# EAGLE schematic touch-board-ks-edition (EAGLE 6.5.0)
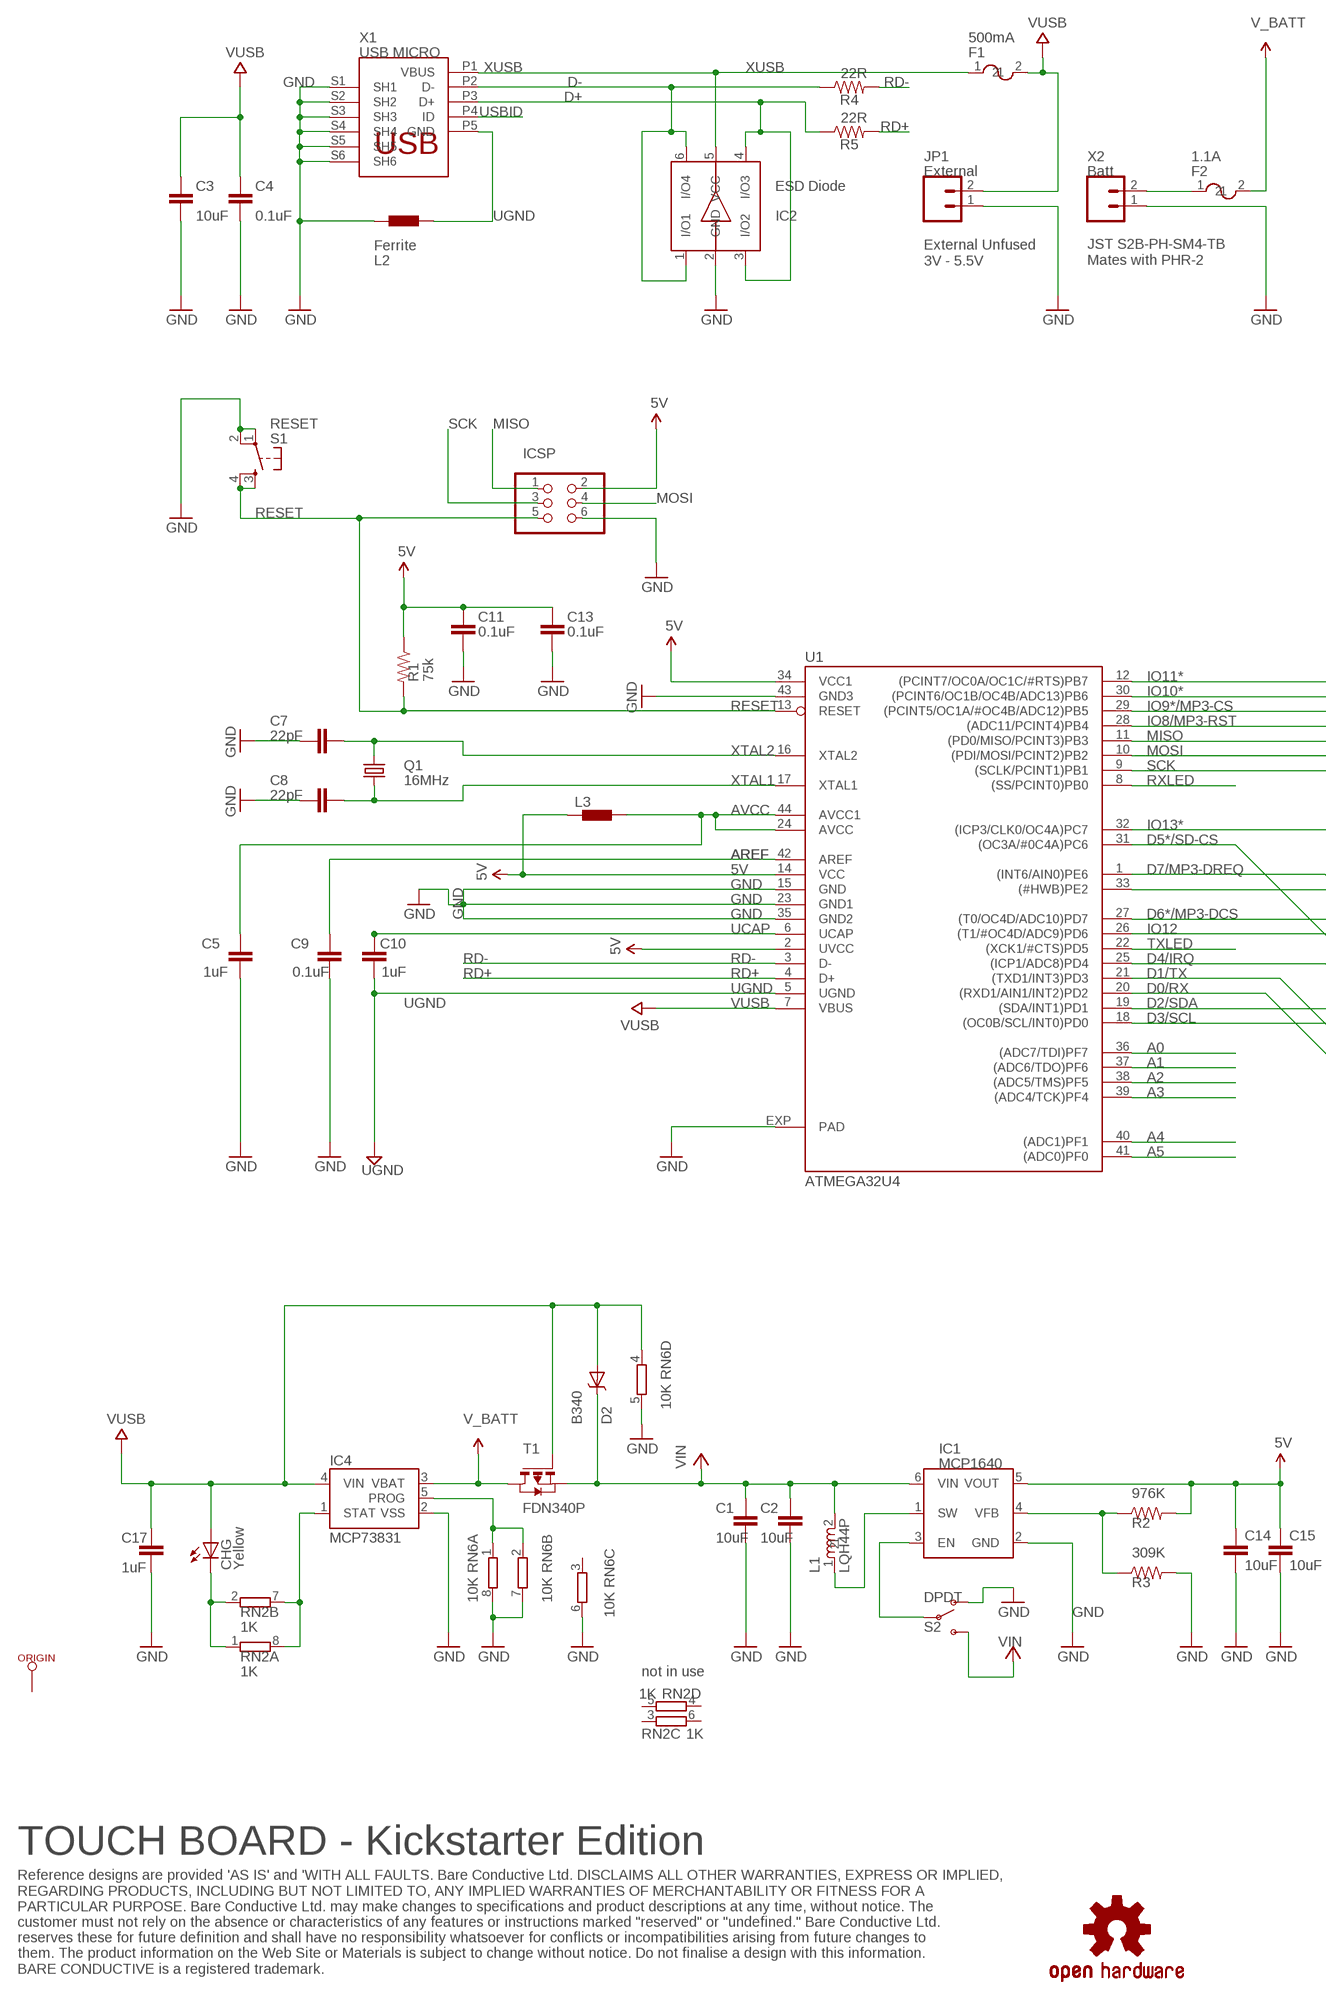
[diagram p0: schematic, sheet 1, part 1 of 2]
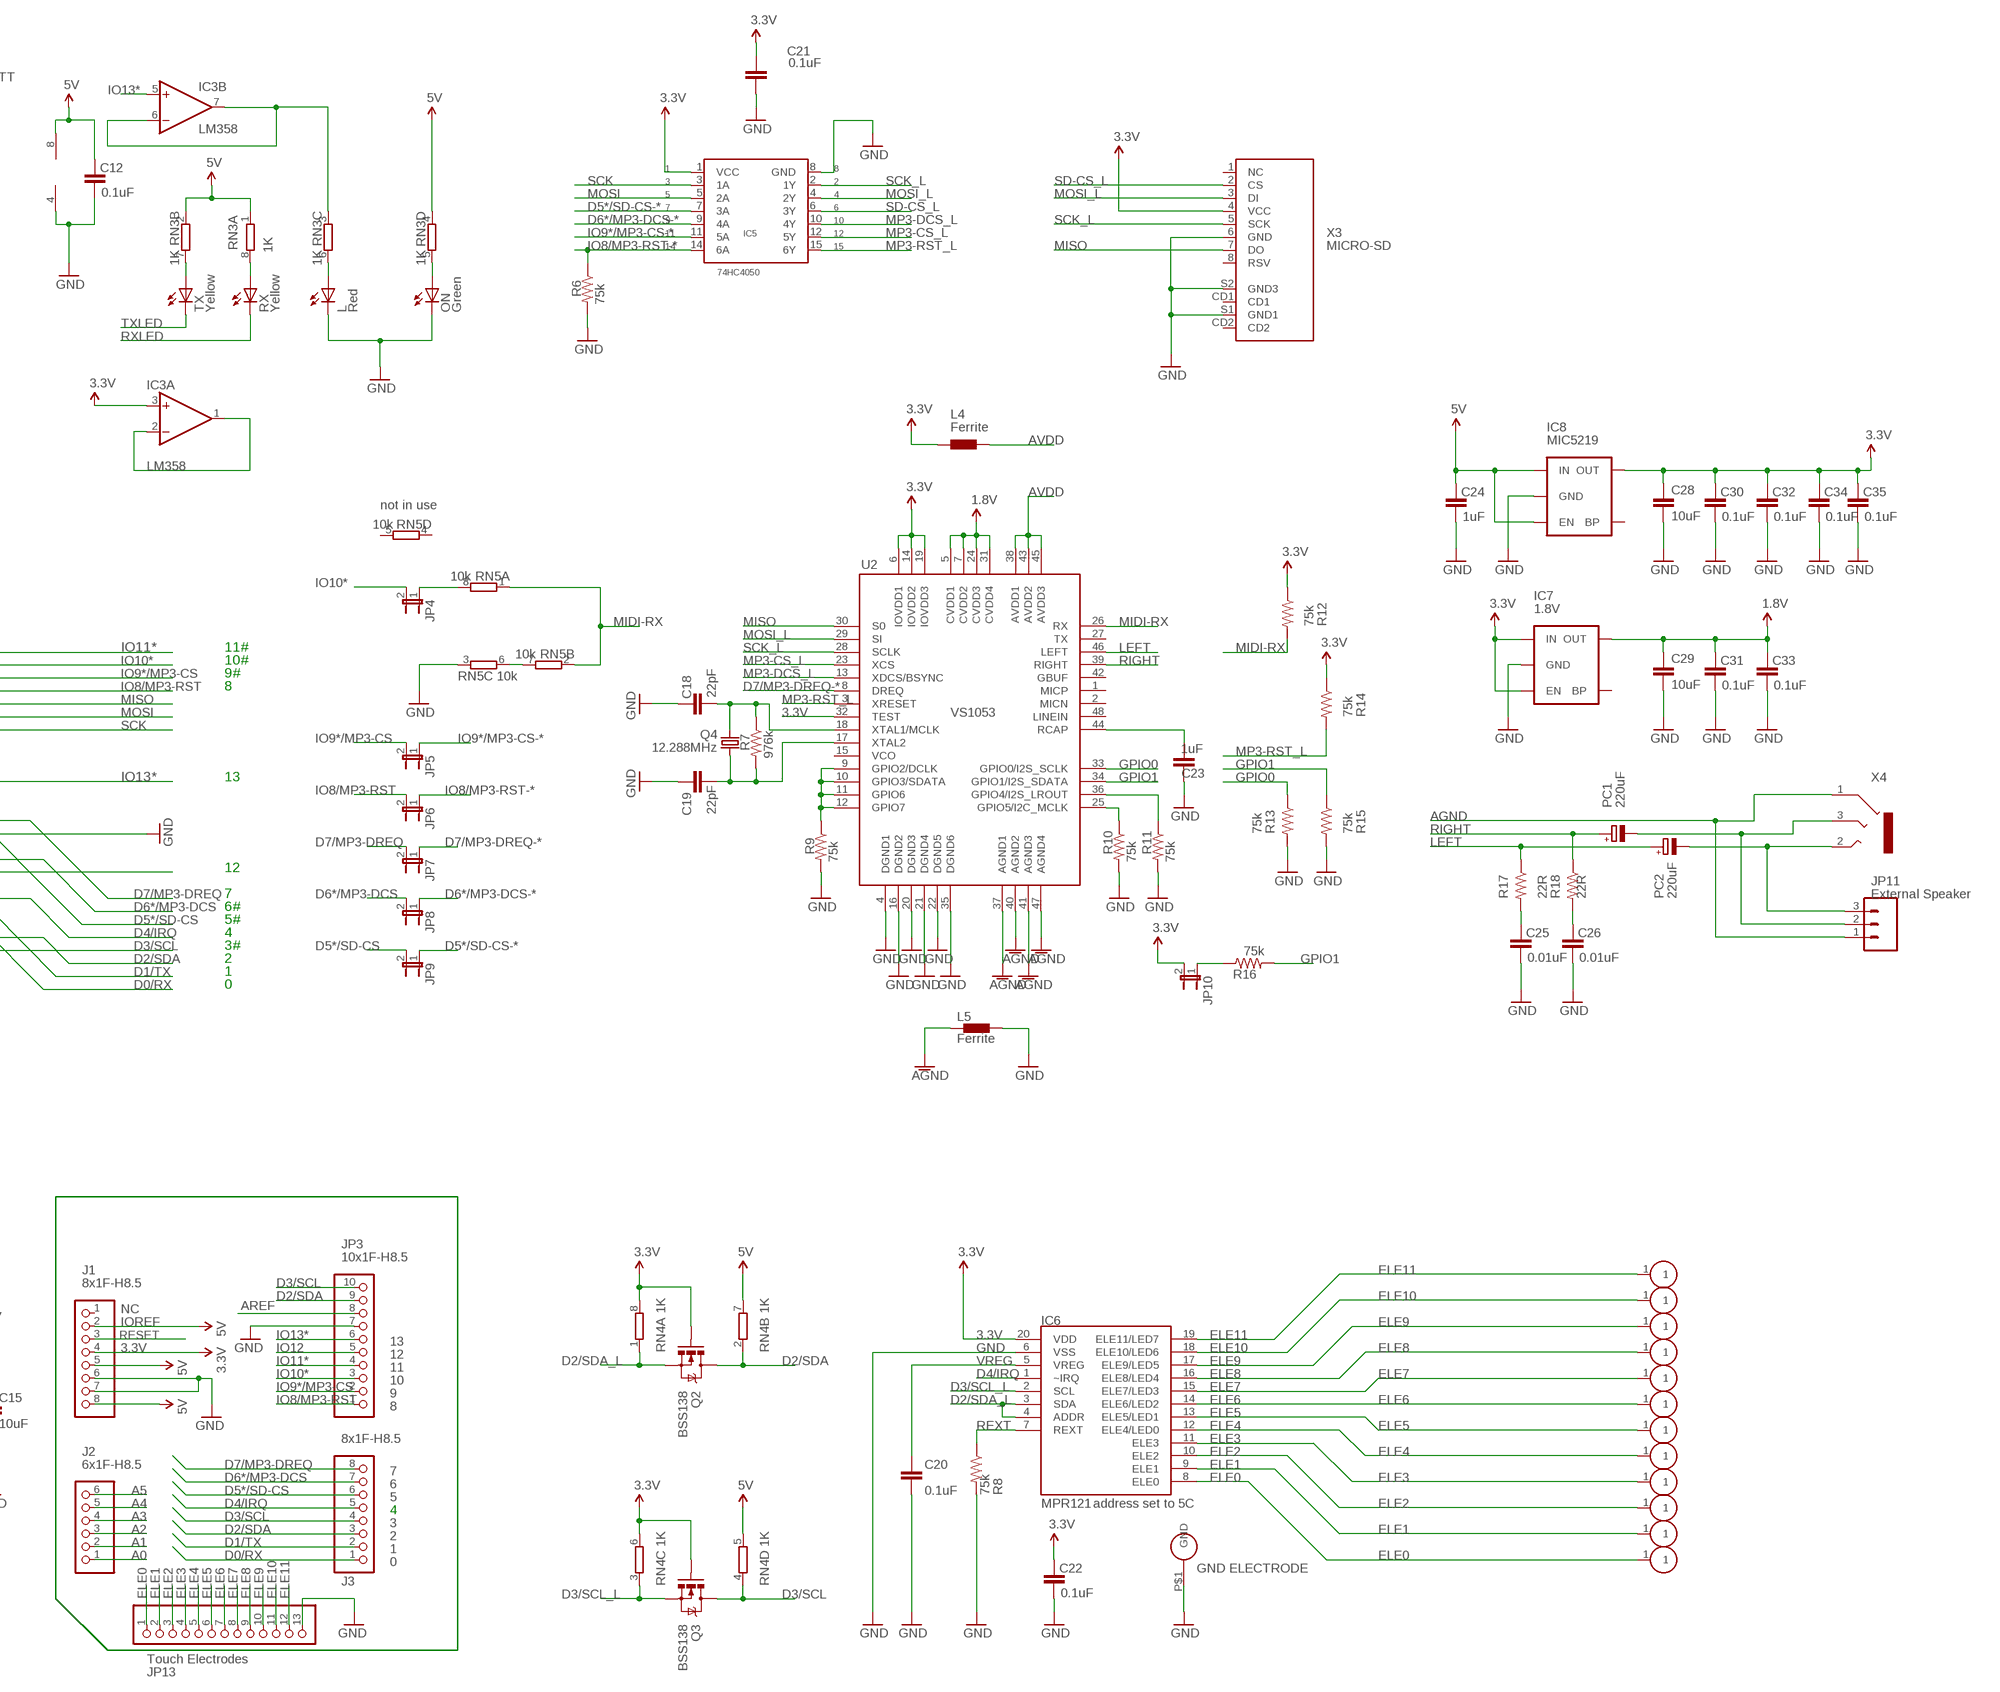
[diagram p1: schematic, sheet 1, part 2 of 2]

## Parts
C1  10uF  CAP1206  [1206]
C2  10uF  CAP1206  [1206]
C3  10uF  CAP1206  [1206]
C4  0.1uF  CAP0402-CAP  [0402-CAP]
C5  1uF  CAP0402-CAP  [0402-CAP]
C7  22pF  CAP0402-CAP  [0402-CAP]
C8  22pF  CAP0402-CAP  [0402-CAP]
C9  0.1uF  CAP0402-CAP  [0402-CAP]
C10  1uF  CAP0402-CAP  [0402-CAP]
C11  0.1uF  CAP0402-CAP  [0402-CAP]
C12  0.1uF  CAP0402-CAP  [0402-CAP]
C13  0.1uF  CAP0402-CAP  [0402-CAP]
C14  10uF  CAP1206  [1206]
C15  10uF  CAP1206  [1206]
C17  1uF  CAP0402-CAP  [0402-CAP]
C18  22pF  CAP0402-CAP  [0402-CAP]
C19  22pF  CAP0402-CAP  [0402-CAP]
C20  0.1uF  CAP0402-CAP  [0402-CAP]
C21  0.1uF  CAP0402-CAP  [0402-CAP]
C22  0.1uF  CAP0402-CAP  [0402-CAP]
C23  1uF  CAP0402-CAP  [0402-CAP]
C24  1uF  CAP0402-CAP  [0402-CAP]
C25  0.01uF  CAP0402-CAP  [0402-CAP]
C26  0.01uF  CAP0402-CAP  [0402-CAP]
C28  10uF  CAP1206  [1206]
C29  10uF  CAP1206  [1206]
C30  0.1uF  CAP0402-CAP  [0402-CAP]
C31  0.1uF  CAP0402-CAP  [0402-CAP]
C32  0.1uF  CAP0402-CAP  [0402-CAP]
C33  0.1uF  CAP0402-CAP  [0402-CAP]
C34  0.1uF  CAP0402-CAP  [0402-CAP]
C35  0.1uF  CAP0402-CAP  [0402-CAP]
CHG  Yellow  LEDCHIPLED_0805  [CHIPLED_0805]
D2  B340  DIODE-SCHOTTKY_  [SMA-DIODE]
F1  500mA  PTC  [0805]
F2  1.1A  PTC  [0805]
IC1  MCP1640  BOOST-REG  [6-LEAD-SOT23]
IC2  ESD Diode  PRTR5V  [SOT457]
IC3  LM358  LMV358MMX  [MSOP08]
IC4  MCP73831  [SOT23-5]
IC5  74HC4050  74HC4050PW  [TSSOP-16]
IC6  MPR121  MPR121QFN20  [QFN-20-0.4MM]
IC7  1.8V  V_REG_LDOSMD2  [SC70]
IC8  MIC5219  V_REG_LDOSMD  [SOT23-5]
ICSP  ICSP  PINHD-2X3  [2X03]
J1  8x1F-H8.5  PINHD-1X8  [1X08]
J2  6x1F-H8.5  PINHD-1X6  [1X06]
J3  8x1F-H8.5  PINHD-1X8  [1X08]
JP1  External  M02PTH  [1X02]
JP3  10x1F-H8.5  PINHD-1X10  [1X10]
JP4  JUMPER-2SMD-NO  [SJ_2S-NO]
JP5  JUMPER-2SMD-NC  [SJ_2S]
JP6  JUMPER-2SMD-NC  [SJ_2S]
JP7  JUMPER-2SMD-NC  [SJ_2S]
JP8  JUMPER-2SMD-NC  [SJ_2S]
JP9  JUMPER-2SMD-NC  [SJ_2S]
JP10  JUMPER-2SMD-NO  [SJ_2S-NO]
JP11  External Speaker  M03PTH  [1X03]
JP13  Touch Electrodes  PINHD-1X13  [1X13]
L  Red  LEDCHIPLED_0805  [CHIPLED_0805]
L1  LQH44P  [LQH44PN100MP0L]
L2  Ferrite  BLM15HB121SN1  [0402]
L3  BLM15HB121SN1  [0402]
L4  Ferrite  BLM15HB121SN1  [0402]
L5  Ferrite  BLM15HB121SN1  [0402]
ON  Green  LEDCHIPLED_0805  [CHIPLED_0805]
ORIGIN  TP_SP  [TP-SP]
PC1  220uF  CPOL-EUD  [PANASONIC_D]
PC2  220uF  CPOL-EUD  [PANASONIC_D]
Q1  16MHz  CRYSTAL5X3  [CRYSTAL-SMD-5X3]
Q2  BSS138  MOSFET-NCHANNELSMD  [SOT23-3]
Q3  BSS138  MOSFET-NCHANNELSMD  [SOT23-3]
Q4  12.288MHz  CRYSTAL5X3  [CRYSTAL-SMD-5X3]
R1  75k  RESISTOR0402-RES  [0402-RES]
R2  976K  RESISTOR0402-RES  [0402-RES]
R3  309K  RESISTOR0402-RES  [0402-RES]
R4  22R  RESISTOR0402-RES  [0402-RES]
R5  22R  RESISTOR0402-RES  [0402-RES]
R6  75k  RESISTOR0402-RES  [0402-RES]
R7  976k  RESISTOR0402-RES  [0402-RES]
R8  75k  RESISTOR0402-RES  [0402-RES]
R9  75k  RESISTOR0402-RES  [0402-RES]
R10  75k  RESISTOR0402-RES  [0402-RES]
R11  75k  RESISTOR0402-RES  [0402-RES]
R12  75k  RESISTOR0402-RES  [0402-RES]
R13  75k  RESISTOR0402-RES  [0402-RES]
R14  75k  RESISTOR0402-RES  [0402-RES]
R15  75k  RESISTOR0402-RES  [0402-RES]
R16  75k  RESISTOR0402-RES  [0402-RES]
R17  22R  RESISTOR0402-RES  [0402-RES]
R18  22R  RESISTOR0402-RES  [0402-RES]
RN2  1K  4R-NCAY16  [CAY16]
RN3  1K  4R-NCAY16  [CAY16]
RN4  1K  4R-NCAY16  [CAY16]
RN5  10k  4R-NCAY16  [CAY16]
RN6  10K  4R-NCAY16  [CAY16]
RX  Yellow  LEDCHIPLED_0805  [CHIPLED_0805]
S1  RESET  TAC_SWITCHSND  [TACTILE_SWITCH_SMD@1]
S2  DPDT  DPDT-SWITCH  [JS202011SCQN]
T1  FDN340P  PMOSSOT23  [SOT-23]
TX  Yellow  LEDCHIPLED_0805  [CHIPLED_0805]
U1  ATMEGA32U4  ATMEGA32U4-XUMU  [QFN44ML7X7]
U2  VS1053  VS1033  [LQFP-48]
U$1  EDGE-ELEC-LEFT  [EDGE-ELEC-LEFT]
U$3  EDGE-ELEC-RIGHT  [EDGE-ELEC-RIGHT]
U$6  EDGE-GND  [EDGE-GND]
U$8  OSHW-LOGO  [OSHW-LOGO]
U$17  EDGE-ELEC  [EDGE-ELEC]
U$18  EDGE-ELEC  [EDGE-ELEC]
U$22  EDGE-ELEC  [EDGE-ELEC]
U$24  EDGE-ELEC  [EDGE-ELEC]
U$26  EDGE-ELEC  [EDGE-ELEC]
U$27  EDGE-ELEC  [EDGE-ELEC]
U$28  EDGE-ELEC  [EDGE-ELEC]
U$29  EDGE-ELEC  [EDGE-ELEC]
U$30  EDGE-ELEC  [EDGE-ELEC]
U$31  EDGE-ELEC  [EDGE-ELEC]
X1  USB MICRO  MYCON2_USB-MINI-B  [CON2_USB_MICRO_B_AT]
X2  Batt  M02-JST-2MM-SMT  [JST-2-SMD]
X3  MICRO-SD  TOBY-SD  [MSDC-PP-02]
X4  SJ-3523  [3POLE-JACK]

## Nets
1.8V: C29.1 C31.2 C33.2 IC7.5(OUT) U2.5(CVDD1) U2.7(CVDD2) U2.24(CVDD3) U2.31(CVDD4)
3.3V: C21.2 C22.2 C28.1 C30.2 C32.2 C34.2 C35.2 IC3.3(A:+IN) IC5.1(VCC) IC6.20(VDD) IC7.1(IN) IC7.3(EN) IC8.5(OUT) J1.4 JP10.2 L4.1 Q2.1(G) Q3.1(G) R12.1 R14.1 RN4.6 RN4.8 U2.6(IOVDD1) U2.14(IOVDD2) U2.19(IOVDD3) U2.32(TEST) X3.4(VCC)
5V: C11.2 C12.2 C13.2 C14.1 C15.1 C24.2 IC1.5(VOUT) IC3.8(P:V+) IC8.1(IN) IC8.3(EN) ICSP.2 J1.2 J1.5 J1.8 L3.1 R1.1 R2.2 RN3.1 RN3.2 RN3.4 RN4.5 RN4.7 U1.2(UVCC) U1.14(VCC) U1.34(VCC1)
A0: J2.1 U1.36((ADC7/TDI)PF7)
A1: J2.2 U1.37((ADC6/TDO)PF6)
A2: J2.3 U1.38((ADC5/TMS)PF5)
A3: J2.4 U1.39((ADC4/TCK)PF4)
A4: J2.5 U1.40((ADC1)PF1)
A5: J2.6 U1.41((ADC0)PF0)
AGND: JP11.1 L5.1 U2.37(AGND1) U2.40(AGND2) U2.41(AGND3) U2.47(AGND4) X4.1
AREF [aref]: C9.2 JP3.8 U1.42(AREF)
AVCC: C5.2 L3.2 U1.24(AVCC) U1.44(AVCC1)
AVDD: L4.2 U2.38(AVDD1) U2.43(AVDD2) U2.45(AVDD3)
D0/RX: J3.1 U1.20((RXD1/AIN1/INT2)PD2)
D1/TX: J3.2 U1.21((TXD1/INT3)PD3)
D2/SDA: J3.3 JP3.9 Q2.3(D) RN4.2 U1.19((SDA/INT1)PD1)
D2/SDA_L: IC6.3(SDA) IC6.4(ADDR) Q2.2(S) RN4.1
D3/SCL: J3.4 JP3.10 Q3.3(D) RN4.4 U1.18((OC0B/SCL/INT0)PD0)
D3/SCL_L: IC6.2(SCL) Q3.2(S) RN4.3
D4/IRQ: IC6.1(~IRQ) J3.5 U1.25((ICP1/ADC8)PD4)
D5*/SD-CS: J3.6 JP9.2 U1.31((OC3A/#0C4A)PC6)
D5*/SD-CS-*: IC5.7(3A) JP9.1
D6*/MP3-DCS: J3.7 JP8.2 U1.27((T0/OC4D/ADC10)PD7)
D6*/MP3-DCS-*: IC5.9(4A) JP8.1
D7/MP3-DREQ: J3.8 JP7.2 U1.1((INT6/AIN0)PE6)
D7/MP3-DREQ-*: JP7.1 U2.8(DREQ)
D+: IC2.3(I/O2) IC2.4(I/O3) R5.1 X1.P3(D+)
D-: IC2.1(I/O1) IC2.6(I/O4) R4.1 X1.P2(D-)
ELE0: IC6.8(ELE0) JP13.1 U$1.1
ELE1: IC6.9(ELE1) JP13.2 U$31.1
ELE2: IC6.10(ELE2) JP13.3 U$30.1
ELE3: IC6.11(ELE3) JP13.4 U$29.1
ELE4: IC6.12(ELE4/LED0) JP13.5 U$28.1
ELE5: IC6.13(ELE5/LED1) JP13.6 U$27.1
ELE6: IC6.14(ELE6/LED2) JP13.7 U$26.1
ELE7: IC6.15(ELE7/LED3) JP13.8 U$24.1
ELE8: IC6.16(ELE8/LED4) JP13.9 U$22.1
ELE9: IC6.17(ELE9/LED5) JP13.10 U$18.1
ELE10: IC6.18(ELE10/LED6) JP13.11 U$17.1
ELE11: IC6.19(ELE11/LED7) JP13.12 U$3.1
G1: R9.1 U2.9(GPIO2/DCLK) U2.10(GPIO3/SDATA) U2.11(GPIO6) U2.12(GPIO7)
G2: R10.1 U2.25(GPIO5/I2C_MCLK)
GND [gnd]: C1.2 C2.2 C3.2 C4.1 C5.1 C7.2 C8.2 C9.1 C11.1 C12.1 C13.1 C14.2 C15.2 C17.1 C18.2 C19.2 C20.1 C21.1 C22.1 C23.2 C24.1 C25.1 C26.1 C28.2 C29.2 C30.1 C31.1 C32.1 C33.1 C34.1 C35.1 IC1.2(GND) IC2.2(GND) IC3.4(P:V-) IC4.2(VSS) IC5.8(GND) IC6.6(VSS) IC7.2(GND) IC8.2(GND) ICSP.6 J1.6 J1.7 JP1.1 JP3.7 JP13.13 L2.1 L5.2 L.C ON.C R3.2 R6.2 R8.2 R9.2 R10.2 R11.2 R13.2 R15.2 RN5.3 RN6.5 RN6.6 RN6.7 RN6.8 S1.1 S1.2 S2.4 U1.15(GND) U1.23(GND1) U1.33((#HWB)PE2) U1.35(GND2) U1.43(GND3) U1.EXP(PAD) U2.4(DGND1) U2.16(DGND2) U2.20(DGND3) U2.21(DGND4) U2.22(DGND5) U2.35(DGND6) U$6.P$1(GND) X1.S1(SH1) X1.S2(SH2) X1.S3(SH3) X1.S4(SH4) X1.S5(SH5) X1.S6(SH6) X2.1 X3.6(GND) X3.S1(GND1) X3.S2(GND3)
GPIO0: R13.1 U2.33(GPIO0/I2S_SCLK)
GPIO1: R15.1 R16.2 U2.34(GPIO1/I2S_SDATA)
IO8/MP3-RST: JP3.1 JP6.2 U1.28((ADC11/PCINT4)PB4)
IO8/MP3-RST-*: IC5.14(6A) JP6.1 R6.1
IO9*/MP3-CS: JP3.2 JP5.2 U1.29((PCINT5/OC1A/#OC4B/ADC12)PB5)
IO9*/MP3-CS-*: IC5.11(5A) JP5.1
IO10*: JP3.3 JP4.2 U1.30((PCINT6/OC1B/OC4B/ADC13)PB6)
IO11*: JP3.4 U1.12((PCINT7/OC0A/OC1C/#RTS)PB7)
IO12: JP3.5 U1.26((T1/#OC4D/ADC9)PD6)
IO13*: IC3.5(B:+IN) JP3.6 U1.32((ICP3/CLK0/OC4A)PC7)
LEFT: PC2.+ R17.1 U2.46(LEFT)
MIDI-RX: R12.2 RN5.1 RN5.2 U2.26(RX)
MISO: ICSP.1 U1.11((PD0/MISO/PCINT3)PB3) U2.30(S0) X3.7(DO)
MOSI: IC5.5(2A) ICSP.4 U1.10((PDI/MOSI/PCINT2)PB2)
MOSI_L: IC5.4(2Y) U2.29(SI) X3.3(DI)
MP3-CS_L: IC5.12(5Y) U2.23(XCS)
MP3-DCS_L: IC5.10(4Y) U2.13(XDCS/BSYNC)
MP3-RST_L: IC5.15(6Y) R14.2 U2.3(XRESET)
N$1: IC3.6(B:-IN) IC3.7(B:OUT) RN3.3
N$2: L.A RN3.6
N$3: RN3.7 TX.A
N$4 [gnd]: IC4.1(STAT) RN2.7 RN2.8
N$5: C23.1 U2.44(RCAP)
N$6: RN3.8 RX.A
N$8: ON.A RN3.5
N$9: C18.1 Q4.3 R7.1 U2.18(XTAL1/MCLK)
N$10: C19.1 Q4.1 R7.2 U2.17(XTAL2)
N$11: IC1.1(SW) L1.1
N$12: IC1.4(VFB) R2.1 R3.1
N$13: F2.1 X2.2
N$14: JP4.1 RN5.8
N$15: IC3.1(A:OUT) IC3.2(A:-IN)
N$19: IC4.5(PROG) RN6.1 RN6.2
N$21: C25.2 R17.2
N$22: C26.2 R18.2
N$23: IC1.3(EN) S2.5
N$24: JP11.3 PC2.- X4.2
N$25: JP10.1 R16.1
N$26: JP11.2 PC1.- X4.3
N$27: RN5.6 RN5.7
N$32: CHG.C RN2.1 RN2.2
N$73: R11.1 U2.36(GPIO4/I2S_LROUT)
RD+: R5.2 U1.4(D+)
RD-: R4.2 U1.3(D-)
RESET: ICSP.5 J1.3 R1.2 S1.3 S1.4 U1.13(RESET)
REXT: IC6.7(REXT) R8.1
RIGHT: PC1.+ R18.1 U2.39(RIGHT)
RXLED: RX.C U1.8((SS/PCINT0)PB0)
SCK: IC5.3(1A) ICSP.3 U1.9((SCLK/PCINT1)PB1)
SCK_L: IC5.2(1Y) U2.28(SCLK) X3.5(SCK)
SD-CS_L: IC5.6(3Y) X3.2(CS)
TXLED: TX.C U1.22((XCK1/#CTS)PD5)
UCAP: C10.2 U1.6(UCAP)
UGND [gnd]: C10.1 L2.2 U1.5(UGND) X1.P5(GND)
USBID: X1.P4(ID)
V_BATT: F2.2 IC4.3(VBAT) T1.1(D)
VCC: C1.1 C2.1 D2.C IC1.6(VIN) L1.2 S2.6 T1.2(S) ; supply symbol labelled VIN
VREG: C20.2 IC6.5(VREG)
VUSB: C3.1 C4.2 C17.2 CHG.A D2.A F1.2 IC4.4(VIN) JP1.2 RN6.4 T1.3(G) U1.7(VBUS)
XTAL1: C8.1 Q1.1 U1.17(XTAL1)
XTAL2: C7.1 Q1.3 U1.16(XTAL2)
XUSB [usbvcc]: F1.1 IC2.5(VCC) X1.P1(VBUS)
Unconnected: IC7.4(BP) IC8.4(BP) J1.1 ORIGIN.X(TESTP) RN2.3 RN2.4 RN2.5 RN2.6 RN5.4 RN5.5 RN6.3 U2.1(MICP) U2.2(MICN) U2.15(VCO) U2.27(TX) U2.42(GBUF) U2.48(LINEIN) X3.1(NC) X3.8(RSV) X3.CD1 X3.CD2

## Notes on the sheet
- USB
- External Unfused
  3V - 5.5V
- JST S2B-PH-SM4-TB
  Mates with PHR-2
- not in use
- 11#
- 10#
- 9#
- 8
- 13
- 12
- 7
- 6#
- 5#
- 4
- 3#
- 2
- 1
- 0
- NC
- IOREF
- 13
- 12
- 11
- 10
- 9
- 8
- 7
- 6
- 5
- address set to 5C
- 4
- not in use
- 3
- 2
- 1
- 0
- GND ELECTRODE
- TOUCH BOARD - Kickstarter Edition
- Reference designs are provided 'AS IS' and 'WITH ALL FAULTS. Bare Conductive Ltd. DISCLAIMS ALL OTHER WARRANTIES, EXPRESS OR IMPLIED,
  REGARDING PRODUCTS, INCLUDING BUT NOT LIMITED TO, ANY IMPLIED WARRANTIES OF MERCHANTABILITY OR FITNESS FOR A 
  PARTICULAR PURPOSE. Bare Conductive Ltd. may make changes to specifications and product descriptions at any time, without notice. The 
  customer must not rely on the absence or characteristics of any features or instructions marked "reserved" or "undefined." Bare Conductive Ltd.
  reserves these for future definition and shall have no responsibility whatsoever for conflicts or incompatibilities arising from future changes to 
  them. The product information on the Web Site or Materials is subject to change without notice. Do not finalise a design with this information.
  BARE CONDUCTIVE is a registered trademark.

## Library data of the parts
C1-C3 C14 C15 C28 C29 = SparkFun-Capacitors:CAP: Capacitor
C4 C5 C7-C13 C17-C26 C30-C35 = SparkFun:CAP: Capacitor
CHG L ON RX TX = led:LED: LED
D2 = SparkFun-DiscreteSemi:DIODE-SCHOTTKY: Commonly MBRA140.; PROD_ID: DIO-09886
F1 F2 = BareConductive:PTC: PTC FUSE 0805
IC1 = BareConductive:BOOST-REG: 0.65V Start-up Synchronous Boost Regulator MCP1640
IC2 = BareConductive:PRTR5V: ESD DIODE
IC3 = linear:LMV358?*: Dual General Purpose, Low Voltage, Rail-to-Rail Output Operational Amplifiers Source: http://www.national.com/mpf/LM/LMV321.html http://www.national.com/dt/lmv_qual.pdf
IC4 = SparkFun:MCP73831: Microchip's MCP73831 Miniature single cell, fully integrated Li-Ion, Li-polymer charge management controller http://ww1.microchip.com/downloads/en/DeviceDoc/21984a.pdf
IC5 = BareConductiveLbr:74HC4050PW
IC6 = SparkFun:MPR121: MPR121 Capacitive Touch Sensor Controller
IC7 IC8 = SparkFun:V_REG_LDO: Voltage Regulator LDO Standard 150mA LDO voltage regulator in SOT-23 layout. Micrel part MIC5205. BP (by-pass) pin is used to lower output noise with 470pF cap.
ICSP = SmartPrj:PINHD-2X3: PIN HEADER
J1 J3 = SmartPrj:PINHD-1X8: PIN HEADER
J2 = SmartPrj:PINHD-1X6: PIN HEADER
JP1 X2 = SparkFun:M02: Header 2
JP3 = SmartPrj:PINHD-1X10: PIN HEADER
JP4-JP10 = SparkFun-Passives:JUMPER-2: Jumper
JP11 = SparkFun:M03: Header 3 Standard 3-pin 0.1" header. Use with straight break away headers (SKU : PRT-00116), right angle break away headers (PRT-00553), swiss pins (PRT-00743), machine pins (PRT-00117), and female headers (PRT-00115). Molex polarized connector foot print use with SKU : PRT-08232 with associated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
JP13 = pinhead:PINHD-1X13: PIN HEADER
L1 = BareConductive:LQH44P: LQH44P CHIP INDUCTOR
L2-L5 = inductors:BLM15H: EMIFIL (R) Chip Ferrite Bead for GHz Noise
ORIGIN = SmartPrj:TP_SP
PC1 PC2 = rcl:CPOL-EU: POLARIZED CAPACITOR, European symbol
Q1 Q4 = SparkFun:CRYSTAL: Crystals
Q2 Q3 = SparkFun:MOSFET-NCHANNEL
R1-R18 = SparkFun:RESISTOR: Resistor
RN2-RN6 = resistor-dil:4R-N: Array Chip Resistor Source: RS Component / Phycomp
S1 = SparkFun:TAC_SWITCH: Momentary Switch Button commonly used for reset or general input. Spark Fun Electronics SKU : COM-00097
S2 = BareConductive:DPDT-SWITCH: JS202011SCQN SLIDE SWITCH
T1 = zetex:PMOSSOT23: MOS FET
U1 = SmartPrj:ATMEGA32U4-XU
U2 = SparkFun:VS1033
U$1 = BareConductiveLbr:EDGE-ELEC-LEFT
U$3 = BareConductiveLbr:EDGE-ELEC-RIGHT
U$6 = BareConductiveLbr:EDGE-GND
U$8 = BareConductive:OSHW-LOGO
U$17 U$18 U$22 U$24 U$26-U$31 = BareConductiveLbr:EDGE-ELEC
X1 = SmartPrj:MYCON2_USB-MINI-B
X3 = BareConductive:TOBY-SD: TOBY MICRO SD CARD HOLDER
X4 = BareConductive:SJ-3523

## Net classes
1 power: width 0.254 mm, drill 0.61 mm, clearance 0.254 mm
2 gnd: width 0.254 mm, drill 0.61 mm, clearance 0.254 mm
3 usbvcc: width 0.254 mm, drill 0.61 mm, clearance 0.254 mm
4 aref: width 0.254 mm, drill 0.61 mm, clearance 0.254 mm

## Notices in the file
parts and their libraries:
SparkFun-Aesthetics: Licensing: CC v3.0 Share-Alike You are welcome to use this library for commercial purposes.
